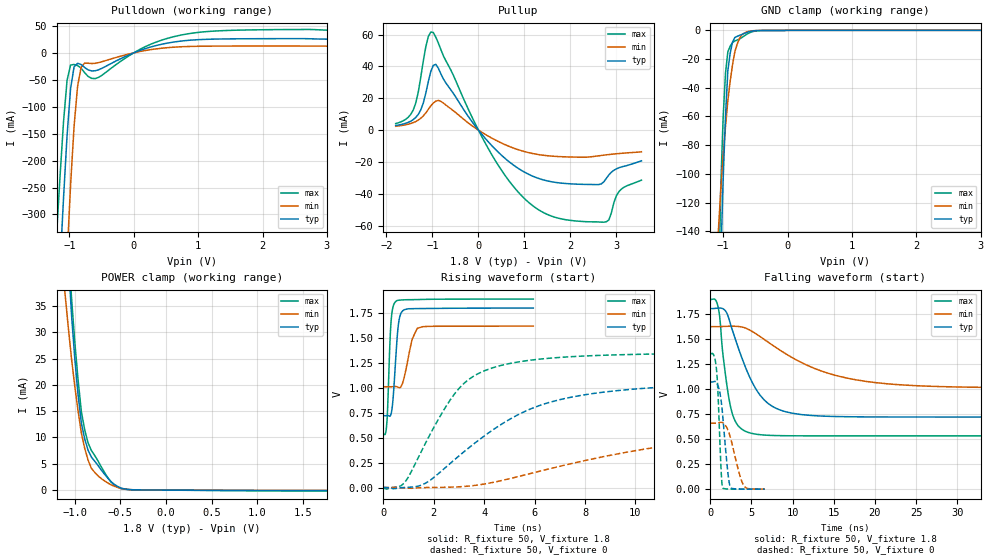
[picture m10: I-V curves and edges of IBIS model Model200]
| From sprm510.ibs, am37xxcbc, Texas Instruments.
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| Model based on original model for DSIPHY_WIO_CORE_GPIOWRAPPER
|   Sub model FBPB_HS00L01_PU1_1P8
[model]   Model200
|[Input Load]   PU
|[Output Drive] SC00LB01
|Voltage   1.8V
|Mode   I/O
Model_type   I/O
Polarity   Non-Inverting
Enable   Active-Low
Vinl =  0.63
Vinh =  1.17
Cref =  15pF
Rref =  100.0000M
Vref =  0V
Vmeas =  0.9
C_comp   1.429432p   1.270657p   1.602015p
[Model Spec]
Vinl   0.63   0.567   0.6615
Vinh   1.17   1.053   1.2285
[Temperature Range]   25   125   -40
[Voltage Range]   1.8   1.62   1.89
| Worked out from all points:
|   slope of the pulldown table from 0 to 0.27 V, typ, clamps not added: 24.3 ohm
|   slope of the pullup table from 0 to 0.27 V, typ, clamps not added: 29.7 ohm
|   GND clamp passes 1 mA (typ) near -0.60 V on its own axis
|   POWER clamp passes 1 mA (typ) near -0.56 V on its own axis
|   rising waveform, R_fixture 50, V_fixture 1.8: 20-80 % time 176ps typ, 308ps min, 123ps max; typ from 0.72 V to 1.8 V
|   rising waveform, R_fixture 50, V_fixture 0: 20-80 % time 4.08ns typ, 9.39ns min, 2.05ns max; typ from 0.001 V to 1.07 V
|   falling waveform, R_fixture 50, V_fixture 1.8: 20-80 % time 3.38ns typ, 8.8ns min, 1.25ns max; typ from 1.8 V to 0.72 V
|   falling waveform, R_fixture 50, V_fixture 0: 20-80 % time 715ps typ, 1.21ns min, 411ps max; typ from 1.07 V to 0.002 V
[POWER_clamp]
-1.8V     362.5mA    191.4mA    412.8mA
-1.109V   56.76mA    37.74mA    60.51mA
-1.073V   44.67mA    31.25mA    47.93mA
-1.036V   33.52mA    25.07mA    36.72mA
-1V       25.06mA    19.75mA    28.2mA
-963.6mV  18.11mA    14.99mA    20.91mA
-927.3mV  12.67mA    10.8mA     14.87mA
-890.9mV  9.734mA    7.935mA    11.44mA
-818.2mV  6.293mA    4.153mA    7.536mA
-636.4mV  2.249mA    1.342mA    2.34mA
-418.2mV  128.7uA    129.3uA    104.4uA
1.764V    -96.73uA   -46.48uA   -163.5uA
[Pulldown]
-1.8V     -1.718A    -2.61A     -1.406A
-1.2V     -527.4mA   -844.5mA   -339.9mA
-1.145V   -396mA     -683.1mA   -229.1mA
-1.091V   -269mA     -526.7mA   -127.5mA
-1.036V   -153.6mA   -378.9mA   -51.17mA
-981.8mV  -66.33mA   -245.6mA   -22.67mA
-927.3mV  -26mA      -136.2mA   -21.54mA
-872.7mV  -19.34mA   -61.98mA   -23.69mA
-763.6mV  -27.2mA    -19.05mA   -36.72mA
-545.5mV  -31.39mA   -18.17mA   -45.46mA
872.7mV   23.46mA    11.88mA    35.92mA
3.545V    25.34mA    12.51mA    41.58mA
[Pullup]
-1.8V     2.903mA    2.423mA    4.112mA
-1.418V   6.595mA    4.711mA    12.64mA
-1.255V   12.69mA    7.42mA     33.24mA
-1.091V   30.4mA     13mA       58.69mA
-981.8mV  40.63mA    17.02mA    61.3mA
-818.2mV  35.38mA    18.12mA    50.59mA
272.7mV   -9.179mA   -4.728mA   -14.55mA
1.255V    -29.75mA   -15.09mA   -48.97mA
2.564V    -34.17mA   -16.31mA   -57.57mA
2.782V    -30.25mA   -15.5mA    -57.48mA
3.055V    -23.63mA   -14.68mA   -38.61mA
3.545V    -19.25mA   -13.56mA   -31.41mA
[GND_clamp]
-1.8V     -2.82A     -1.192A    -3.165A
-1.073V   -235.8mA   -138.4mA   -192.1mA
-1.036V   -159.6mA   -110.8mA   -107.6mA
-1V       -103.8mA   -87.86mA   -60.73mA
-963.6mV  -60.04mA   -67.29mA   -29.86mA
-927.3mV  -28.26mA   -49.09mA   -14.98mA
-890.9mV  -15.95mA   -35.49mA   -11.09mA
-854.5mV  -8.198mA   -24.09mA   -8.559mA
-818.2mV  -4.99mA    -14.87mA   -7.387mA
-709.1mV  -2.858mA   -3.093mA   -5.012mA
-527.3mV  -395.6uA   -260.4uA   -751.2uA
3.6V      0A         0A         0A
[Ramp]
dV/dt_f  0.6511198/3.385323n   0.3681672/8.874134n   0.8172568/1.253019n
dV/dt_r  0.6490312/4.094928n   0.399712/9.467846n   0.8198593/2.051071n
R_load = 50
[Rising Waveform]
R_fixture = 50
V_fixture = 1.8
V_fixture_min = 1.62
V_fixture_max = 1.89
0s        720.1mV    1.01V      534.5mV
144ps     721.2mV    1.011V     674.9mV
270ps     717.6mV    1.01V      1.517V
324ps     761.3mV    1.01V      1.719V
513ps     1.386V     1.012V     1.87V
594ps     1.632V     1.004V     1.877V
711ps     1.754V     1.017V     1.88V
1.143ns   1.793V     1.488V     1.883V
1.341ns   1.794V     1.596V     1.884V
5.949ns   1.799V     1.618V     1.89V
[Rising Waveform]
R_fixture = 50
V_fixture = 0
V_fixture_min = 0
V_fixture_max = 0
0s        1.324mV    1.072mV    -5.589mV
837ps     977uV      -4.146mV   47.36mV
1.674ns   43.68mV    -73.7uV    446.2mV
2.52ns    212.9mV    2.997mV    827.8mV
3.357ns   391.3mV    13.94mV    1.078V
4.491ns   602.9mV    59.05mV    1.212V
6.426ns   841.4mV    177.8mV    1.293V
12.55ns   1.025V     463.7mV    1.344V
20.76ns   1.062V     596.8mV    1.35V
60.39ns   1.069V     657.1mV    1.35V
[Falling Waveform]
R_fixture = 50
V_fixture = 1.8
V_fixture_min = 1.62
V_fixture_max = 1.89
0s        1.8V       1.62V      1.89V
621ps     1.802V     1.62V      1.888V
1.044ns   1.805V     1.62V      1.777V
1.872ns   1.774V     1.623V     1.123V
2.682ns   1.585V     1.624V     751.6mV
4.455ns   1.179V     1.6V       571.6mV
6.966ns   858.9mV    1.469V     538.5mV
11.12ns   743.7mV    1.261V     532.9mV
21.29ns   720.5mV    1.052V     532.6mV
44.16ns   720mV      1.012V     532.6mV
[Falling Waveform]
R_fixture = 50
V_fixture = 0
V_fixture_min = 0
V_fixture_max = 0
0s        1.069V     658.8mV    1.35V
468ps     1.074V     658.7mV    1.328V
783ps     1.06V      659.1mV    1.167V
945ps     1.032V     661.4mV    941.8mV
1.341ns   868.7mV    667.7mV    149.4mV
1.503ns   740.6mV    663.8mV    18.15mV
2.142ns   163mV      588.9mV    3.072mV
2.448ns   22.16mV    514.1mV    2.517mV
4.104ns   2.24mV     33.89mV    1.93mV
6.615ns   1.654mV    2.596mV    1.806mV
